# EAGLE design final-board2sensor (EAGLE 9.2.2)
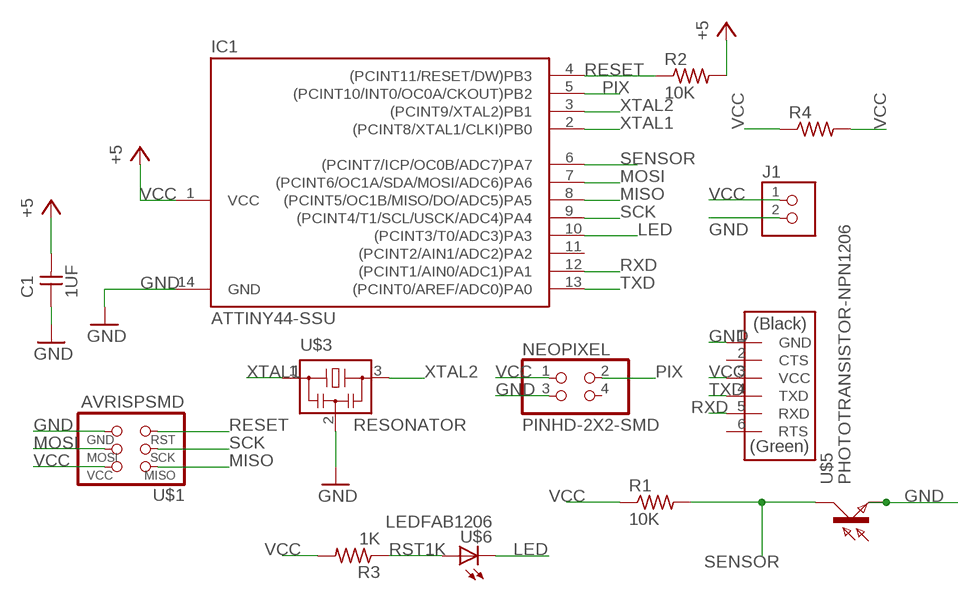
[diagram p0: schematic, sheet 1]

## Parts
C1  1UF  CAP-UNPOLARIZEDFAB  [C1206FAB]
IC1  ATTINY44-SSU  [SOIC14]
J1  TERM-1X02-ADAFRUIT  [3.5MMTERM]
NEOPIXEL  PINHD-2X2-SMD  [2X02SMD]
R1  10K  RES-US1206FAB  [R1206FAB]
R2  10K  RES-US1206FAB  [R1206FAB]
R3  1K  RES-US1206FAB  [R1206FAB]
R4  RES-US1206FAB  [R1206FAB]
U$1  AVRISPSMD  [2X03SMD]
U$2  FTDI-SMD-HEADER  [1X06SMD]
U$3  RESONATOR  [EFOBM]
U$5  PHOTOTRANSISTOR-NPN1206  [OP1206]
U$6  LEDFAB1206  [LED1206FAB]

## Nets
GND: C1.1 IC1.14(GND) J1.2 NEOPIXEL.3 U$1.6(GND) U$2.1(GND) U$3.2 U$5.EMITTER(E)
LED: IC1.10((PCINT3/T0/ADC3)PA3) U$6.2(C)
MISO: IC1.8((PCINT5/OC1B/MISO/DO/ADC5)PA5) U$1.1(MISO)
MOSI: IC1.7((PCINT6/OC1A/SDA/MOSI/ADC6)PA6) U$1.4(MOSI)
PIX: IC1.5((PCINT10/INT0/OC0A/CKOUT)PB2) NEOPIXEL.2
RESET: IC1.4((PCINT11/RESET/DW)PB3) R2.1 U$1.5(RST)
RST1K: R3.1 U$6.1(A)
RXD: IC1.12((PCINT1/AIN0/ADC1)PA1) U$2.5(RXD)
SCK: IC1.9((PCINT4/T1/SCL/USCK/ADC4)PA4) U$1.3(SCK)
SENSOR: IC1.6((PCINT7/ICP/OC0B/ADC7)PA7) R1.2 U$5.COLLECTOR(C)
TXD: IC1.13((PCINT0/AREF/ADC0)PA0) U$2.4(TXD)
VCC: C1.2 IC1.1(VCC) J1.1 NEOPIXEL.1 R1.1 R2.2 R3.2 R4.1 R4.2 U$1.2(VCC) U$2.3(VCC) ; supply symbol labelled +5
XTAL1: IC1.2((PCINT8/XTAL1/CLKI)PB0) U$3.1
XTAL2: IC1.3((PCINT9/XTAL2)PB1) U$3.3
Unconnected: IC1.11((PCINT2/AIN1/ADC2)PA2) NEOPIXEL.4 U$2.2(CTS) U$2.6(RTS)

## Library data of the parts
C1 = fab:CAP-UNPOLARIZED
IC1 = fab:ATTINY44
J1 = fab:TERM-1X02: 3.5mm terminal block, 2 positions ED555-2DS as found in the fablab inventory.
NEOPIXEL = fab:PINHD-2X2-SMD
R1-R4 = fab:RES-US: Resistor (US Symbol)
U$1 = fab:AVRISP
U$2 = fab:FTDI-SMD-HEADER
U$3 = fab:RESONATOR
U$5 = fab:PHOTOTRANSISTOR-NPN
U$6 = fab:LED: LED

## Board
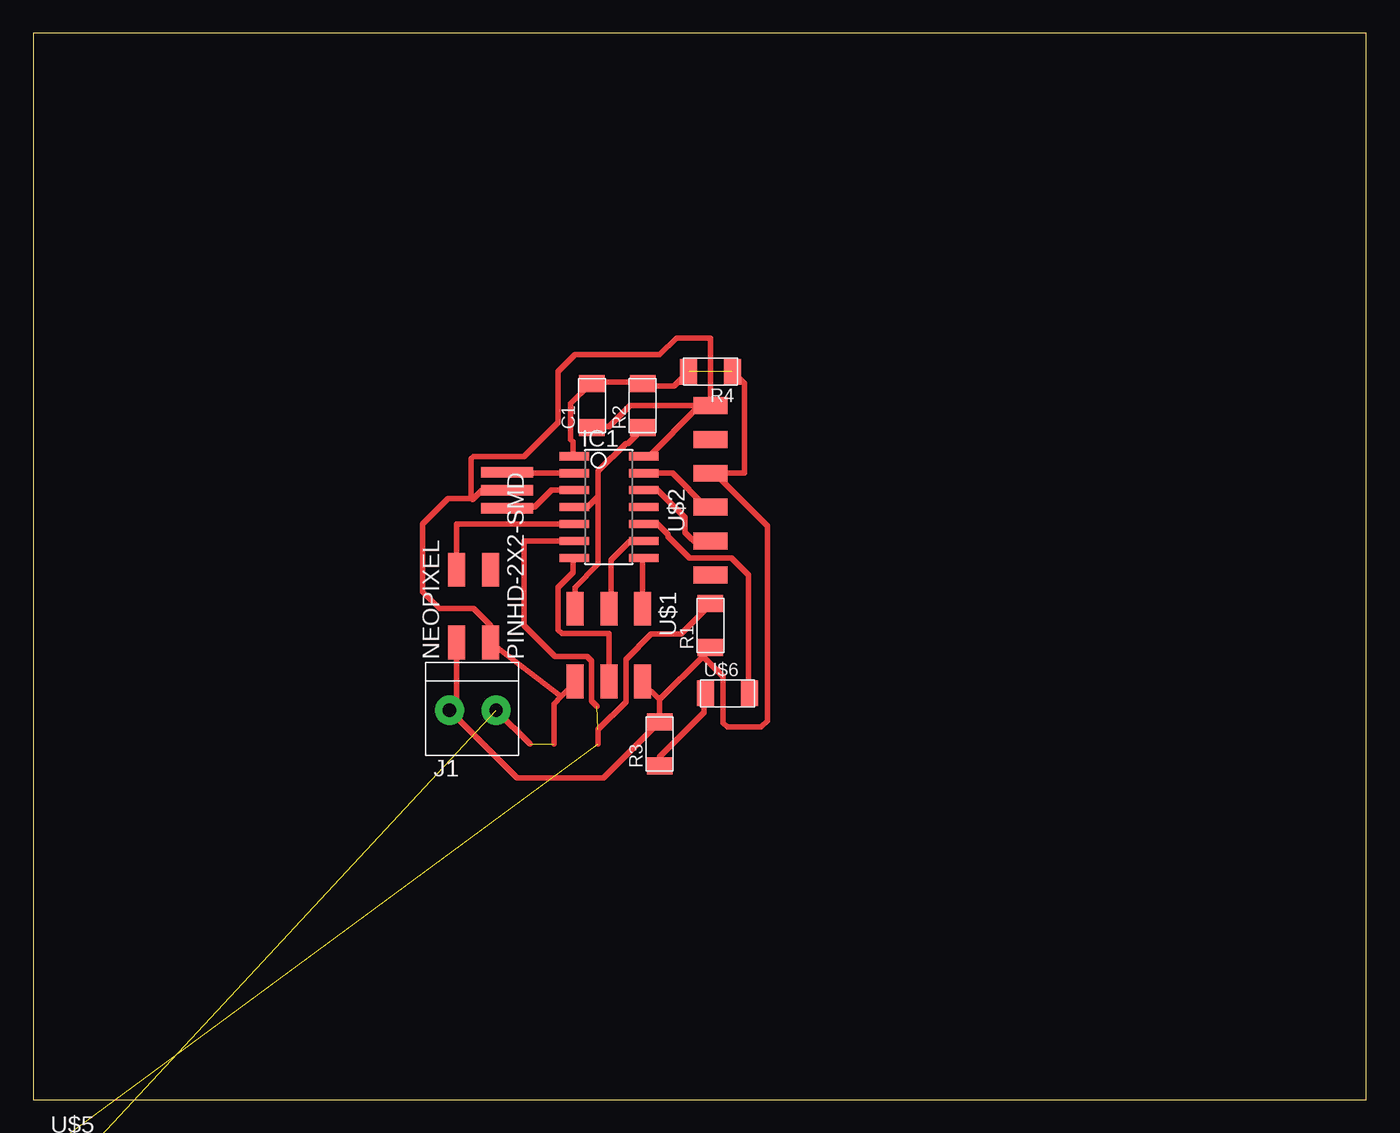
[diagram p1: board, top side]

Size 100 x 80 mm. Coordinates in mm from the lower left corner, seen from the top.
Outline: 0,0 100,0 100,80 0,80 0,0
Copper layers (1*16): Top 0.035mm / dielectric 1.5mm / Bottom 0.035mm
Design rules "rules": minimum track width 16mil, minimum drill 0.8mm, track to track 16mil, track to pad 16mil, pad to pad 16mil, via to via 16mil, smd to smd 16mil, copper to edge 40mil, drill to drill 6mil, minimum pad ring 10mil, minimum via ring 8mil, stop-mask expansion 4mil, vias tented up to drill 0mil, thermal gap 10mil

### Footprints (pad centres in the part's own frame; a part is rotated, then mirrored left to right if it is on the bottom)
C1206FAB = smd 1.27 x 1.905: 1 -1.651,0; 2 1.651,0
SOIC14 = smd 0.61 x 2.21: 1 -3.81,-2.603; 2 -2.54,-2.603; 3 -1.27,-2.603; 4 0,-2.603; 5 1.27,-2.603; 6 2.54,-2.603; 7 3.81,-2.603; 8 3.81,2.603; 9 2.54,2.603; 10 1.27,2.603; 11 0,2.603; 12 -1.27,2.603; 13 -2.54,2.603; 14 -3.81,2.603
3.5MMTERM = drill 1 pad 2.184: 1 1.8,0; 2 -1.7,0
2X02SMD = smd 2.54 x 1.27: 1 -2.54,1.27; 2 2.92,1.27; 3 -2.54,-1.27; 4 2.92,-1.27
R1206FAB = smd 1.27 x 1.905: 1 -1.651,0; 2 1.651,0
2X03SMD = smd 2.54 x 1.27: 1 -2.54,2.54; 2 2.92,2.54; 3 -2.54,0; 4 2.92,0; 5 -2.54,-2.54; 6 2.92,-2.54
1X06SMD = smd 2.54 x 1.27: 1 0,6.35; 2 0,3.81; 3 0,1.27; 4 0,-1.27; 5 0,-3.81; 6 0,-6.35
EFOBM = smd 0.8 x 3.9: 1 -1.35,0; 2 0,0; 3 1.35,0
OP1206 = smd 1.5 x 1.6: COLLECTOR -1.55,0; EMITTER 1.55,0
LED1206FAB = smd 1.27 x 1.905: 1 -1.651,0; 2 1.651,0

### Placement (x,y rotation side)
C1  41.91,52.07 90 top
IC1  43.18,44.45 270 top
J1  33.02,29.21 180 top
NEOPIXEL  33.02,36.83 90 top
R1  50.8,35.56 90 top
R2  45.72,52.07 90 top
R3  46.99,26.67 90 top
R4  50.8,54.61 180 top
U$1  43.18,34.29 270 top
U$2  50.8,45.72 0 top
U$3  35.56,45.72 270 top
U$5  not placed on the board
U$6  52.07,30.48 0 top

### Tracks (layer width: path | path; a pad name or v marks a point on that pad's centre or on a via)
GND  (2 unrouted)
  Top 0.406: U$2.1 44.77,52.07 43.18,50.48 41.91,50.48 C1.1 | IC1.14 46.2,48.26 49.85,51.91 U$2.1 | 39.05,26.67 39.05,29.69 39.61,30.24 | 39.61,30.24 40.64,31.27 U$1.6 | 39.61,30.24 NEOPIXEL.3 34.29,35.56 33.02,36.83 30.48,36.83 29.21,38.1 29.21,43.18 31.11,45.09 32.86,45.09 | U$3.2 33.66,45.72 32.94,45.01 32.86,45.09 | 37.26,26.67 J1.2 | U$2.1 50.8,57.15 48.26,57.15 46.99,55.88 40.64,55.88 39.37,54.61 39.37,50.8 36.83,48.26 33.02,48.26 32.86,48.1 32.86,45.09
LED
  Top 0.406: IC1.10 46.83,43.18 47.62,42.39 47.62,42.23 49.21,40.64 52.39,40.64 53.66,39.37 53.66,30.48 U$6.2
MISO
  Top 0.406: 45.72,40.58 IC1.8 45.72,40.48 U$1.1
MOSI
  Top 0.406: 43.18,31.75 U$1.4 43.18,34.95 39.66,34.95 39.37,35.24 39.37,38.42 40.48,39.53 40.48,40.64 IC1.7
PIX
  Top 0.406: IC1.5 36.83,43.18 36.2,43.18 31.75,43.18 NEOPIXEL.2
RESET
  Top 0.406: 42.39,45.24 42.39,47.15 44.45,49.21 44.61,49.21 45.72,50.32 R2.1 | 42.39,45.24 41.59,44.45 IC1.4 | U$1.5 40.64,38.42 42.39,40.16 42.39,45.24
RST1K
  Top 0.406: R3.1 46.99,25.72 50.32,29.05 50.32,30.48 U$6.1
RXD
  Top 0.406: U$2.5 49.53,41.91 49.53,41.97 49.37,42.07 48.9,42.55 48.9,43.66 46.83,45.72 IC1.12
SCK
  Top 0.406: IC1.9 44.77,41.91 43.34,40.48 43.34,36.99 U$1.3
SENSOR  (2 unrouted)
  Top 0.406: 42.39,26.67 42.39,27.78 44.45,29.84 44.45,33.02 46.35,34.92 48.58,34.92 50.8,37.15 R1.2 | 42.29,29.49 41.88,29.9 41.88,32.89 41.53,33.25 39.37,33.25 39.14,33.25 36.83,35.56 36.83,41.91 IC1.6
TXD
  Top 0.406: IC1.13 47.94,46.99 50.48,44.45 U$2.4
VCC  (1 unrouted)
  Top 0.406: 45.91,53.53 R2.2 45.56,53.82 41.91,53.82 C1.2 41.75,53.66 40.32,52.23 40.32,49.53 40.48,49.37 40.48,48.26 IC1.1 | 45.91,53.53 46.1,53.34 | 46.99,30 R3.2 | 46.99,30 45.72,31.27 U$1.2 | 46.99,30 50.24,33.26 | 50.24,33.26 50.8,33.81 R1.1 | R3.2 46.83,28.26 | 50.24,33.26 51.75,31.75 51.75,28.26 52.07,27.94 54.61,27.94 55.09,28.42 55.09,29.37 55.09,30.48 55.09,43.02 51.12,46.99 U$2.3 53.34,46.99 53.34,53.72 R4.1 | R4.2 48.07,53.53 45.91,53.53 | NEOPIXEL.1 31.75,29.74 J1.1 36.3,24.13 42.8,24.13 R3.2
XTAL1
  Top 0.406: 35.64,46.99 U$3.1 35.72,46.99 IC1.2
XTAL2
  Top 0.406: 35.64,44.45 35.6,44.41 | 35.6,44.41 U$3.3 36.99,44.45 37.62,44.45 38.89,45.72 IC1.3 | 36.83,44.45 36.79,44.41 35.6,44.41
